// single traffic light

(*
	 _
	| |
	|o| red light
	|o| yellow light
	|o| green light
	|_|
	
*)

FUNCTION_BLOCK FB_SingleTrafficLight
VAR_INPUT
	// name
	sInName						: STRING; 	// name of traffic light
	
	// commissioning mode
	bInCommissioning			: BOOL; 	// sensor signal commissioning mode (on rising edge)
	bInRedLightOn				: BOOL;		// test signal to toggle red light state (true/false -> on/off) 
	bInYellowLightOn			: BOOL;		// test signal to toggle yellow light on (true/false -> on/off)
	bInGreenLightOn				: BOOL;		// test signal to toggle green light on (true/false -> on/off)
		
	// automatic mode
	bInAutomatic				: BOOL; 	// sensor signal automatic mode (on rising edge)
	
	// automatic active
	bInAutomaticActive			: BOOL; 	// sensor signal automatic active mode (on rising edge) -> red and green on request

	bInRedRequest				: BOOL;		// sensor signal request red (on rising edge)
	bInGreenRequest				: BOOL;		// sensor signal request green (on rising edge)
	
	// automatic stand by
	bInAutomaticStandBy			: BOOL;		// sensor signal automatic stand by mode (on rising edge) -> yellow light blinks  
	
END_VAR
VAR_OUTPUT
	// lights
	bOutRedLight		AT %Q* 	: BOOL;  	// actor signal red light
	bOutYellowLight		AT %Q* 	: BOOL; 	// actor signal yellow light
	bOutGreenLight		AT %Q* 	: BOOL; 	// actor signal green light
	
	// commissioning mode
	bOutCommissioningMode		: BOOL;		// status signal commissioning mode active
	
	// automatic mode
	bOutAutomaticMode			: BOOL;		// status signal automatic mode active
	bOutAutomaticActiveMode		: BOOL;		// status signal automatic active mode active
	
	// automatic active
	bOutRedRequestReady			: BOOL;		// signal red state reached
	bOutGreenRequestReady		: BOOL;		// signal green state reached
	
END_VAR
VAR
	// commissioning mode
	eOpmodeState				: E_STLOpmodeState;				// opmode state
	fbRTrigInCommissioning		: R_TRIG;						// rising edge detection
	
	// automatic mode
	eAutomaticState				: E_STLAutomaticState;			// automatic state
	fbRTrigInAutomatic			: R_TRIG;						// rising edge detection
	
	// automatic active
	eAutomaticActiveState		: E_STLAutomaticActiveState;	// automatic state
	fbRTrigInAutomaticActive	: R_TRIG;						// rising edge detection
	fbTimerRed					: TON;							// timer for activate red state
	fbTimerYellowRed			: TON;							// timer for activate yellow red state
	fbTimerGreen				: TON;							// timer for activate green state
	fbTimerYellow				: TON;							// timer for activate yellow state
	fbRTrigInRedRequest			: R_TRIG;						// rising edge detection
	fbRTrigInGreenRequest		: R_TRIG;						// rising edge detection 
	
	// automatic stand by
	fbRTrigInAutomaticStandBy	: R_TRIG;						// rising edge detection 
	fbBlinker					: FB_Blinker;					// blinker
	
	// HMI Data
	stHmiData					: ST_STLHmiData;				// hmi data to interaction with hmi
	
END_VAR

METHOD M_Automatic : BOOL
VAR_INPUT
END_VAR
// automatic state machine
CASE eAutomaticState OF

	eSTLAutomatic_StandBy:
		M_AutomaticStandBy();
		IF fbRTrigInAutomaticActive.Q AND NOT fbRTrigInAutomaticStandBy.Q  THEN
			bOutRedRequestReady := FALSE;
			bOutGreenRequestReady := FALSE;
			eAutomaticActiveState := eSTLAutoActive_Red;
			eAutomaticState := eSTLAutomatic_Active;
		END_IF

	eSTLAutomatic_Active:
		M_AutomaticActive();
		IF NOT fbRTrigInAutomaticActive.Q  AND fbRTrigInAutomaticStandBy.Q THEN
			eAutomaticState := eSTLAutomatic_StandBy;			
		END_IF
		
END_CASE
END_METHOD

METHOD M_AutomaticActive : BOOL
VAR_INPUT
END_VAR
// automatic active mode state machine
CASE eAutomaticActiveState OF
	
	// red state and waiting on green request
	eSTLAutoActive_Red:
		bOutRedRequestReady := TRUE;
		bOutGreenRequestReady := FALSE;
	
		fbTimerYellowRed(PT:=T#2S);
		IF fbRTrigInGreenRequest.Q THEN
			fbTimerYellowRed.IN := TRUE;
		END_IF
		IF fbTimerYellowRed.Q THEN
			fbTimerYellowRed(IN:=FALSE);
			eAutomaticActiveState := eSTLAutoActive_YellowRed;
		END_IF
	
	// yellow red state	
	eSTLAutoActive_YellowRed:
		bOutRedRequestReady := FALSE;
		bOutGreenRequestReady := FALSE;
		
		fbTimerGreen(IN:=TRUE,PT:=T#2S);
		IF fbTimerGreen.Q THEN
			fbTimerGreen(IN:=FALSE);
			eAutomaticActiveState := eSTLAutoActive_Green;
		END_IF

	// green state and waiting on red request
	eSTLAutoActive_Green:
		bOutRedRequestReady := FALSE;
		bOutGreenRequestReady := TRUE;	
		
		fbTimerYellow(PT:=T#2S);
		IF fbRTrigInRedRequest.Q THEN
			fbTimerYellow.IN := TRUE;
		END_IF
		IF fbTimerYellow.Q THEN
			fbTimerYellow(IN:=FALSE);
			eAutomaticActiveState := eSTLAutoActive_Yellow;
		END_IF
	
	// yellow state	
	eSTLAutoActive_Yellow:
		bOutRedRequestReady := FALSE;
		bOutGreenRequestReady := FALSE;
		
		fbTimerRed(IN:=TRUE,PT:=T#2S);
		IF fbTimerRed.Q THEN
			fbTimerRed(IN:=FALSE);
			eAutomaticActiveState := eSTLAutoActive_Red;
		END_IF
	
END_CASE
END_METHOD

METHOD M_AutomaticStandBy : BOOL
VAR_INPUT
END_VAR
// reset timers
fbTimerYellowRed(IN:=FALSE);
fbTimerGreen(IN:=FALSE);
fbTimerYellow(IN:=FALSE);
fbTimerRed(IN:=FALSE);
// implement additional functions for automatic stand by mode
END_METHOD

METHOD M_Commissioning : BOOL
VAR_INPUT
END_VAR
// implement additional functions for commissioning mode
END_METHOD

METHOD M_Cycle : BOOL
VAR_INPUT
END_VAR
// process input signals
M_Input();

// opmode state machine
CASE eOpmodeState OF
	
	eSTLOpmode_Commissioning:
		M_Commissioning();
		IF fbRTrigInAutomatic.Q AND NOT fbRTrigInCommissioning.Q THEN
			eAutomaticState := eSTLAutomatic_StandBy;	
			eOpmodeState := eSTLOpmode_Automatic;
		END_IF
		
	eSTLOpmode_Automatic:
		M_Automatic();
		IF NOT fbRTrigInAutomatic.Q AND fbRTrigInCommissioning.Q THEN
			eOpmodeState := eSTLOpmode_Commissioning;
		END_IF

END_CASE

// set output signals
M_Output();
END_METHOD

METHOD M_Input : BOOL
VAR_INPUT
END_VAR
// process input signals

// commissioning mode
fbRTrigInCommissioning(CLK := bInCommissioning OR stHmiData.bInCommissioning);

// automatic mode
fbRTrigInAutomatic(CLK := bInAutomatic OR stHmiData.bInAutomatic);

// automatic Active
fbRTrigInAutomaticActive(CLK := bInAutomaticActive OR stHmiData.bInAutomaticActive);


fbRTrigInRedRequest(CLK := bInRedRequest OR stHmiData.bInAutoActiveRedRequest);
fbRTrigInGreenRequest(CLK := bInGreenRequest OR stHmiData.bInAutoActiveGreenRequest);

// automatic stand by
fbRTrigInAutomaticStandBy(CLK := bInAutomaticStandBy OR stHmiData.bInAutomaticStandBy);
END_METHOD

METHOD M_Output : BOOL
VAR_INPUT
END_VAR
// set output signals

// commissioning mode
IF (eOpmodeState = eSTLOpmode_Commissioning) THEN
	bOutCommissioningMode := TRUE;
ELSE
	bOutCommissioningMode := FALSE;
END_IF

// automatic mode
IF (eOpmodeState = eSTLOpmode_Automatic) THEN
	bOutAutomaticMode := TRUE;
ELSE
	bOutAutomaticMode := FALSE;
END_IF

IF (eAutomaticState = eSTLAutomatic_Active) THEN
	bOutAutomaticActiveMode := TRUE;
ELSE
	bOutAutomaticActiveMode := FALSE;	
END_IF

// red light
IF (eOpmodeState = eSTLOpmode_Automatic AND eAutomaticState = eSTLAutomatic_Active) AND (eAutomaticActiveState = eSTLAutoActive_Red OR eAutomaticActiveState = eSTLAutoActive_YellowRed) 
	OR eOpmodeState = eSTLOpmode_Commissioning AND (bInRedLightOn OR stHmiData.bInCommissioningRedLightOn) THEN
	bOutRedLight := TRUE;
ELSE
	bOutRedLight := FALSE;
END_IF

// yellow light
IF (eOpmodeState = eSTLOpmode_Automatic AND eAutomaticState = eSTLAutomatic_Active)  AND (eAutomaticActiveState = eSTLAutoActive_Yellow OR eAutomaticActiveState = eSTLAutoActive_YellowRed) 
	OR eOpmodeState = eSTLOpmode_Commissioning AND (bInYellowLightOn OR stHmiData.bInCommissioningYellowLightOn) THEN
	fbBlinker(CLK := FALSE);
	bOutYellowLight := TRUE;
ELSIF  eOpmodeState = eSTLOpmode_Automatic AND eAutomaticState = eSTLAutomatic_StandBy THEN
	fbBlinker(CLK := TRUE);
	bOutYellowLight := fbBlinker.Q;
ELSE
	fbBlinker(CLK := FALSE);
	bOutYellowLight := FALSE;
END_IF

// green light
IF (eOpmodeState = eSTLOpmode_Automatic AND eAutomaticState = eSTLAutomatic_Active) AND (eAutomaticActiveState = eSTLAutoActive_Green) 
	OR eOpmodeState = eSTLOpmode_Commissioning AND (bInGreenLightOn OR stHmiData.bInCommissioningGreenLightOn) THEN
	bOutGreenLight := TRUE;
ELSE
	bOutGreenLight := FALSE;
END_IF

// hmi output data
stHmiData.sOutName := sInName;
stHmiData.bOutCommissioningMode := bOutCommissioningMode;
stHmiData.bOutAutomaticMode := bOutAutomaticMode;
stHmiData.bOutAutomaticActiveMode := bOutAutomaticActiveMode;
stHmiData.bOutRedLightStatus := bOutRedLight;
stHmiData.bOutYellowLightStatus := bOutYellowLight;
stHmiData.bOutGreenLightStatus := bOutGreenLight;
END_METHOD

END_FUNCTION_BLOCK
